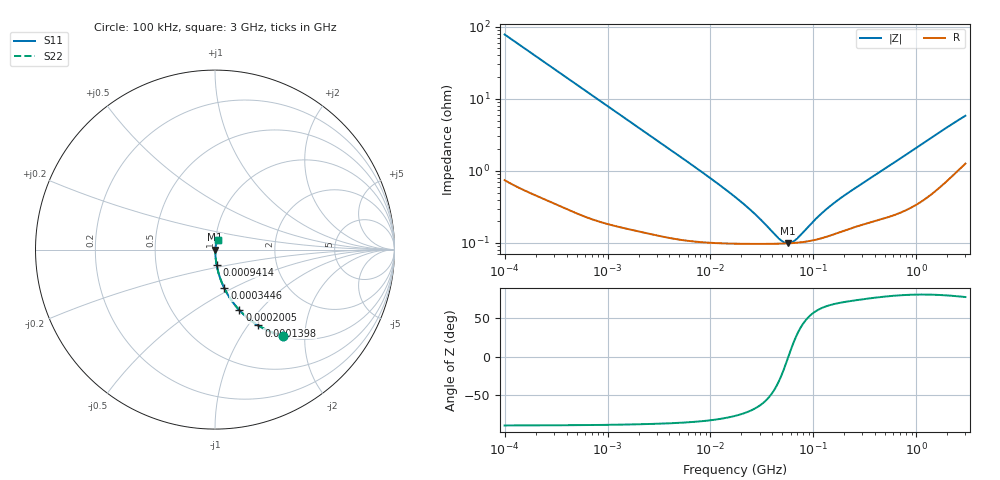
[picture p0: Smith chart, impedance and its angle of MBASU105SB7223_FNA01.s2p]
! MBASU105SB7223_FNA01  S-PARAMETER MODEL  ( Standard Model )
! Model Generated by TAIYO YUDEN Corporation (http://www.ty-top.com)
! Version 2.0
! TAIYO YUDEN Control No. 230906
! Copyright(c) 2014 TAIYO YUDEN CO.,LTD. All Rights Reserved.
! Product Description (link to TY-COMPAS)
! https://ds.yuden.co.jp/TYCOMPAS/or/detail?pn=MBASU105SB7223KFNA01&u=M
! Products Name : Multilayer Ceramic Capacitors
! Characteristics :
!  Capacitance : 0.022 [uF] , Rated Voltage : 50 [V] , TCC : X7R
!  Case Size : 1.0 x 0.5 / 0.039 x 0.02 [mm/inch] , Thickness : 0.5 / 0.02 [mm/inch]
!  (Conditions: Temperature = 25 [degC] , DC Bias Voltage = 0 [V])
! External Node Assignments :
!  1  o---| |---o  2
! GND o---------o GND
! Frequency Range : 100kHz  -  3GHz  [ 401 STEP ]
# MHZ S RI R 50
! Freq[MHz].  S11 Real  S11 Imag  S21 Real  S21 Imag  S12 Real  S12 Imag  S22 Real  S22 Imag
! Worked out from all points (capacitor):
!   401 points, 100 kHz to 3 GHz, reference 50 ohm
!   read as one part in series: C = 20.3 nF near 105.3 kHz
!   lowest |Z| = 98.5 mohm at 56.68 MHz (marker M1)
!   series resonance near 57.19 MHz, so ESL is about 380 pH
!   S11 on the Smith chart (normalised r, x): 100 kHz: 1.01, -1.56; 139.8 kHz: 1.01, -1.12; 200.5 kHz: 1.01, -0.78; 344.6 kHz: 1.01, -0.46; 941.4 kHz: 1.00, -0.17; 3 GHz: 1.03, +0.11
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0.1  0.3809 -0.4809  0.6191 0.4809  0.6191 0.4809  0.3809 -0.4809
0.1398  0.2414 -0.4228  0.7586 0.4228  0.7586 0.4228  0.2414 -0.4228
0.200542  0.1358 -0.3368  0.8642 0.3368  0.8642 0.3368  0.1358 -0.3368
0.259498  0.087 -0.2756  0.913 0.2756  0.913 0.2756  0.087 -0.2756
0.344552  0.0525 -0.216  0.9475 0.216  0.9475 0.216  0.0525 -0.216
0.562235  0.0216 -0.1372  0.9784 0.1372  0.9784 0.1372  0.0216 -0.1372
0.941399  0.00887 -0.0833  0.9911 0.0833  0.9911 0.0833  0.00887 -0.0833
3.161081  0.00189 -0.0252  0.9981 0.0252  0.9981 0.0252  0.00189 -0.0252
9.093698  0.00108 -0.00864  0.9989 0.00864  0.9989 0.00864  0.00108 -0.00864
17.7727  0.000989 -0.00411  0.999 0.00411  0.999 0.00411  0.000989 -0.00411
27.54426  0.000971 -0.00226  0.999 0.00226  0.999 0.00226  0.000971 -0.00226
47.32384  0.000974 -0.000541  0.999 0.000541  0.999 0.000541  0.000974 -0.000541
52.46276  0.000979 -0.000245  0.999 0.000245  0.999 0.000245  0.000979 -0.000245
56.67997  0.000984 -2.53e-05  0.999 2.53e-05  0.999 2.53e-05  0.000984 -2.53e-05
61.23616  0.00099 0.000195  0.999 -0.000195  0.999 -0.000195  0.00099 0.000195
67.88584  0.001 0.00049  0.999 -0.00049  0.999 -0.00049  0.001 0.00049
97.38194  0.00108 0.00158  0.9989 -0.00158  0.9989 -0.00158  0.00108 0.00158
129.3002  0.0012 0.00254  0.9988 -0.00254  0.9988 -0.00254  0.0012 0.00254
176.1623  0.0014 0.00374  0.9986 -0.00374  0.9986 -0.00374  0.0014 0.00374
547.5153  0.00243 0.0115  0.9976 -0.0115  0.9976 -0.0115  0.00243 0.0115
1838.476  0.00781 0.0362  0.9922 -0.0362  0.9922 -0.0362  0.00781 0.0362
3000  0.0155 0.0553  0.9845 -0.0553  0.9845 -0.0553  0.0155 0.0553
